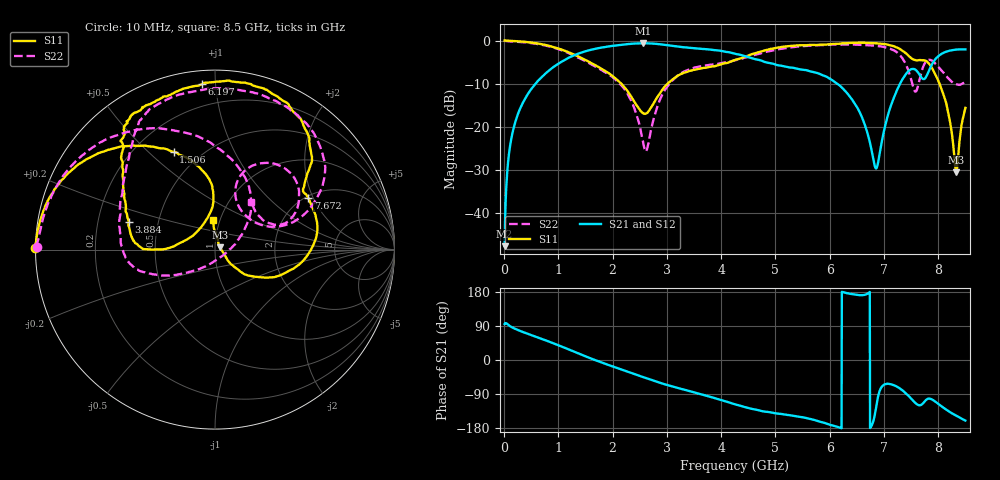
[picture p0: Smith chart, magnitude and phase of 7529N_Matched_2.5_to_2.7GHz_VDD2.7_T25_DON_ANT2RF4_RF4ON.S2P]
!Agilent Technologies,E5071C,MY46417908,A.11.23
!Date: Wed Oct 16 15:59:31 2019
!Data & Calibration Information:
!Freq	S11:SOLT2(ON)	S21:SOLT2(ON)	S12:SOLT2(ON)	S22:SOLT2(ON)
!PortZ  Port1:50+j0  Port2:50+j0
!Above PortZ is port z conversion or system Z0 setting when saving the data.
!When reading, reference impedance value at option line is always used.
# Hz S dB R 50
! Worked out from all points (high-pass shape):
!   1601 points, 10 MHz to 8.5 GHz, reference 50 ohm
!   highest |S21| = -0.62 dB at 2.568 GHz (marker M1); lowest = -47.7 dB at 10 MHz (marker M2)
!   |S21| within 3 dB of the highest: 1.252 GHz to 4.438 GHz (3.185 GHz wide, 112 % of centre); 8.001 GHz to end of sweep
!   lowest |S11| = -30.6 dB at 8.33 GHz (marker M3), VSWR 1.06, Z = 52.7 + j1.37 ohm
!   |S11| at or under -10 dB: 2.159 GHz to 3.013 GHz (854.5 MHz wide, 33 % of centre); 8.023 GHz to end of sweep
!   |S22| runs from -25.8 to 0.0 dB; largest |S21 - S12| = 0.0066
!   S11 on the Smith chart (normalised r, x): 10 MHz: -0.00, +0.00; 1.506 GHz: 0.36, +0.60; 3.884 GHz: 0.34, +0.14; 6.197 GHz: 0.07, +0.92; 7.672 GHz: 2.07, +1.84; 8.5 GHz: 0.93, +0.31
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1e7  0.01 179.5  -47.70 95.1  -47.76 94.9  -0.05 179.0
1.055125e8  -0.04 175.2  -24.89 89.7  -24.90 89.8  -0.19 173.7
3.0715e8  -0.21 166.3  -15.48 76.1  -15.53 76.2  -0.36 162.9
9.0145e8  -1.46 140.7  -6.23 44.4  -6.30 44.6  -1.60 129.4
1.426769e9  -4.04 116.5  -2.78 13.9  -2.80 14.0  -4.31 94.5
1.506362e9  -4.57 113.0  -2.45 9.4  -2.49 9.4  -4.84 89.5
2.228012e9  -10.95 91.8  -0.88 -28.4  -0.90 -28.4  -11.43 43.8
2.567612e9  -16.85 128.1  -0.62 -45.5  -0.63 -45.5  -23.98 -17.8
2.843538e9  -12.75 175.5  -0.82 -58.9  -0.81 -59.0  -14.62 -138.4
3.883562e9  -5.94 162.1  -2.21 -100.7  -2.19 -100.8  -5.52 172.7
4.255e9  -4.49 148.0  -3.05 -116.9  -3.08 -117.3  -4.57 152.9
5.671769e9  -1.03 116.4  -7.23 -156.7  -7.18 -156.7  -1.16 108.7
6.197088e9  -0.68 94.6  -10.57 -178.9  -10.59 -179.3  -0.94 84.2
6.568525e9  -0.51 80.8  -17.08 171.0  -17.11 170.8  -1.01 66.4
6.849756e9  -0.61 71.4  -29.65 -129.4  -29.73 -129.2  -1.22 54.8
7.088538e9  -1.03 61.2  -16.61 -62.9  -16.68 -62.7  -1.79 43.4
7.4812e9  -3.85 37.9  -6.77 -98.9  -6.80 -99.0  -8.20 19.6
7.672225e9  -4.52 28.8  -8.26 -119.2  -8.26 -119.4  -8.11 71.9
7.879169e9  -6.24 -8.4  -5.64 -103.7  -5.65 -103.9  -4.62 39.0
8.091419e9  -12.38 -37.4  -2.87 -125.4  -2.88 -125.4  -7.37 20.8
8.3302e9  -30.58 26.1  -2.08 -147.3  -2.08 -147.1  -10.12 34.1
8.5e9  -15.62 93.9  -2.05 -159.8  -2.02 -159.7  -9.57 52.6
